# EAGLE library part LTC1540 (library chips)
LTC Nanopower Comparator with Bandgap reference
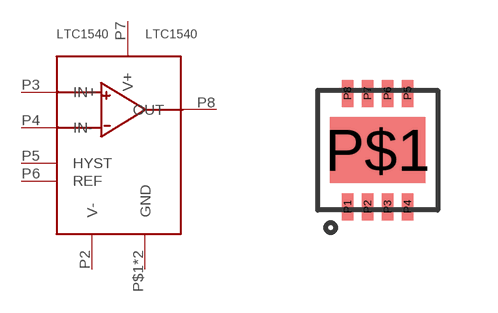
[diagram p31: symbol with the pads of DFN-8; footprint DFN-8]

Designator prefix -

## LTC1540 (DIGIKEY: LTC1540CDD#PBF-ND)  [DFN-8]
P1  GND
P2  V-
P3  IN+
P4  IN-
P5  HYST
P6  REF
P7  V+
P8  OUT
P$1  GND

## Footprint DFN-8 (pad centres in mm)
smd 0.28 x 0.675: P1 -0.75,-1.42; P2 -0.25,-1.42; P3 0.25,-1.42; P4 0.75,-1.42; P5 0.75,1.42; P6 0.25,1.42; P7 -0.25,1.42; P8 -0.75,1.42
smd 2.38 x 1.65: P$1 0,0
